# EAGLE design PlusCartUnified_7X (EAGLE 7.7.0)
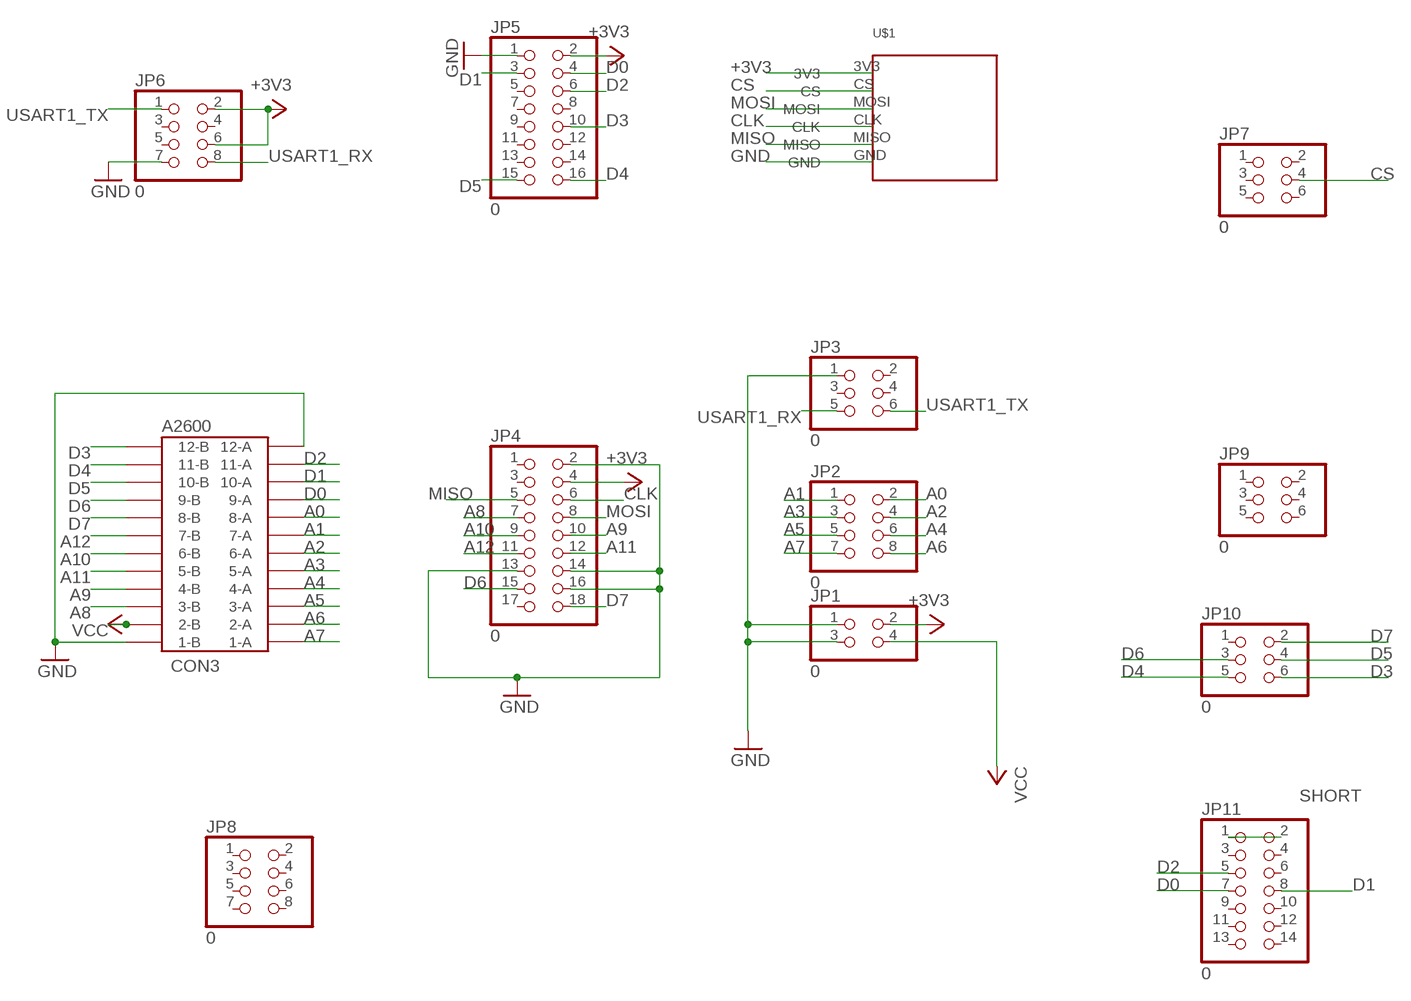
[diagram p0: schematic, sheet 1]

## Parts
CON3  A2600  24PINEDGE-254MM  [24PINEDGE-254MM]
JP1  0  PINHD-2X2  [2X02]
JP2  0  PINHD-2X4  [2X04]
JP3  0  PINHD-2X3  [2X03]
JP4  0  PINHD-2X9  [2X09]
JP5  0  PINHD-2X8  [2X08]
JP6  0  PINHD-2X4  [2X04]
JP7  0  PINHD-2X3  [2X03]
JP8  0  PINHD-2X4  [2X04]
JP9  0  PINHD-2X3  [2X03]
JP10  0  PINHD-2X3  [2X03]
JP11  0  PINHD-2X7  [2X07]
U$1  MICROSD2MICROSD2  [MICROSD_FOOTPRINT]

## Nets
+3V3: JP1.2 JP4.4 JP5.2 JP6.2 JP6.6 U$1.3V3
A0: CON3.8-A JP2.2
A1: CON3.7-A JP2.1
A2: CON3.6-A JP2.4
A3: CON3.5-A JP2.3
A4: CON3.4-A JP2.6
A5: CON3.3-A JP2.5
A6: CON3.2-A JP2.8
A7: CON3.1-A JP2.7
A8: CON3.3-B JP4.7
A9: CON3.4-B JP4.10
A10: CON3.6-B JP4.9
A11: CON3.5-B JP4.12
A12: CON3.7-B JP4.11
CLK: JP4.6 U$1.CLK
CS: JP7.4 U$1.CS
D0: CON3.9-A JP5.4 JP11.7
D1: CON3.10-A JP5.3 JP11.8
D2: CON3.11-A JP5.6 JP11.5
D3: CON3.12-B JP5.10 JP10.6
D4: CON3.11-B JP5.16 JP10.5
D5: CON3.10-B JP5.15 JP10.4
D6: CON3.9-B JP4.15 JP10.3
D7: CON3.8-B JP4.18 JP10.2
GND: CON3.1-B CON3.12-A JP1.1 JP1.3 JP3.1 JP4.2 JP4.13 JP4.14 JP4.16 JP5.1 JP6.7 U$1.GND
MISO: JP4.5 U$1.MISO
MOSI: JP4.8 U$1.MOSI
SHORT: JP11.1 JP11.2
USART1_RX: JP3.5 JP6.8
USART1_TX: JP3.6 JP6.1
VCC: CON3.2-B JP1.4
Unconnected: JP3.2 JP3.3 JP3.4 JP4.1 JP4.3 JP4.17 JP5.5 JP5.7 JP5.8 JP5.9 JP5.11 JP5.12 JP5.13 JP5.14 JP6.3 JP6.4 JP6.5 JP7.1 JP7.2 JP7.3 JP7.5 JP7.6 JP8.1 JP8.2 JP8.3 JP8.4 JP8.5 JP8.6 JP8.7 JP8.8 JP9.1 JP9.2 JP9.3 JP9.4 JP9.5 JP9.6 JP10.1 JP11.3 JP11.4 JP11.6 JP11.9 JP11.10 JP11.11 JP11.12 JP11.13 JP11.14

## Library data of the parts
CON3 = con-edge:24PINEDGE-254MM: 24 PIN EDGE CONNECTOR 2.54mm ATARI 2600 CARTRIDGE PORT
JP1 = pinhead:PINHD-2X2: PIN HEADER
JP2 JP6 = pinhead:PINHD-2X4: PIN HEADER
JP3 = pinhead:PINHD-2X3: PIN HEADER
JP4 = pinhead:PINHD-2X9: PIN HEADER
JP5 = pinhead:PINHD-2X8: PIN HEADER
JP7 JP9 JP10 = pinhead@1:PINHD-2X3: PIN HEADER
JP8 = pinhead@1:PINHD-2X4: PIN HEADER
JP11 = pinhead@1:PINHD-2X7: PIN HEADER
U$1 = MICROSD:MICROSD2

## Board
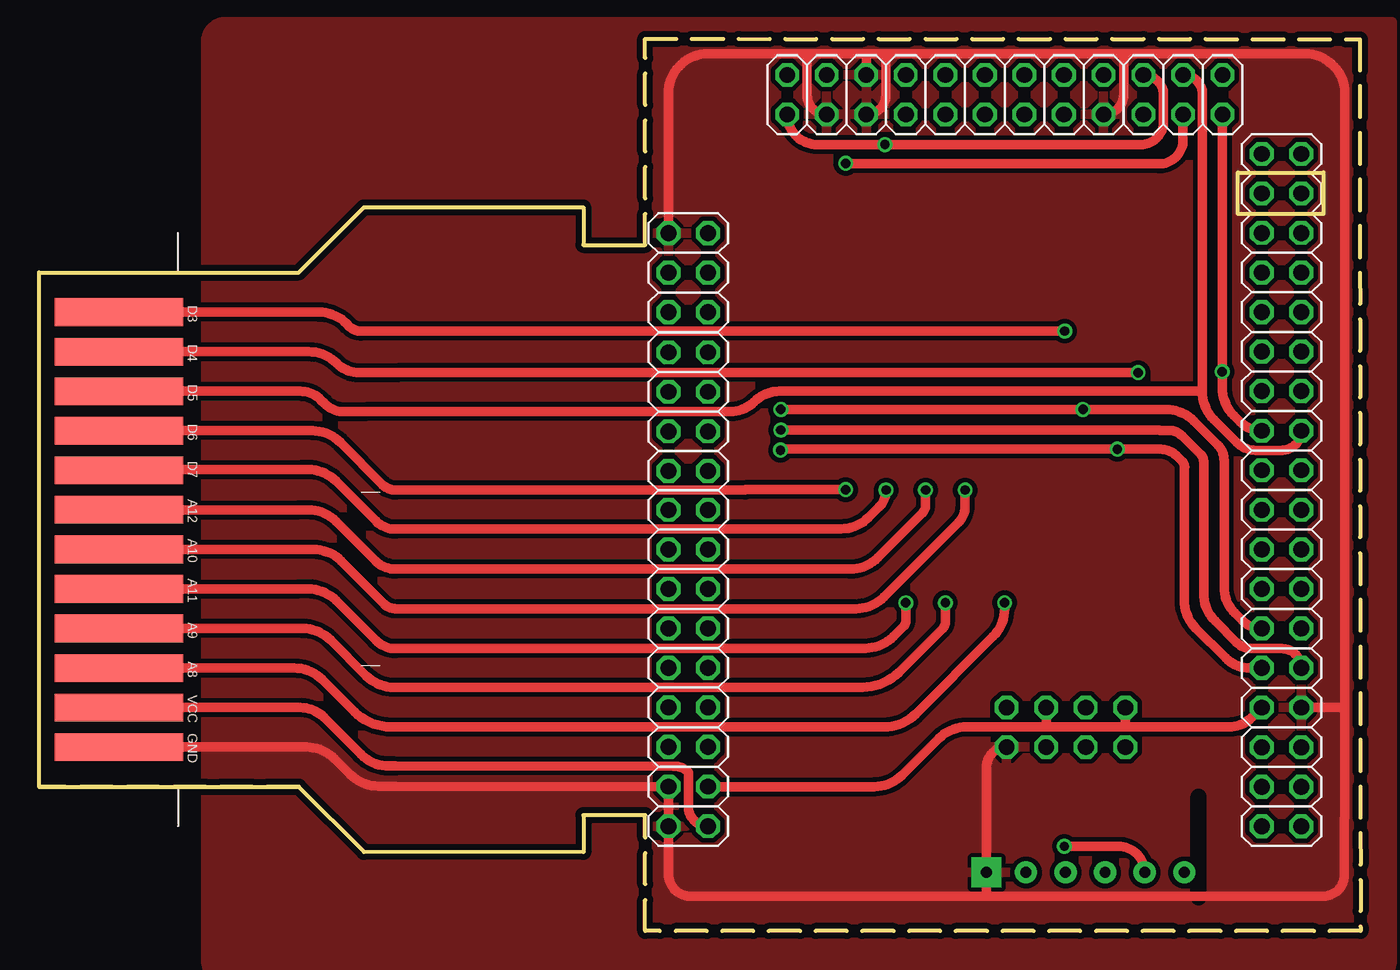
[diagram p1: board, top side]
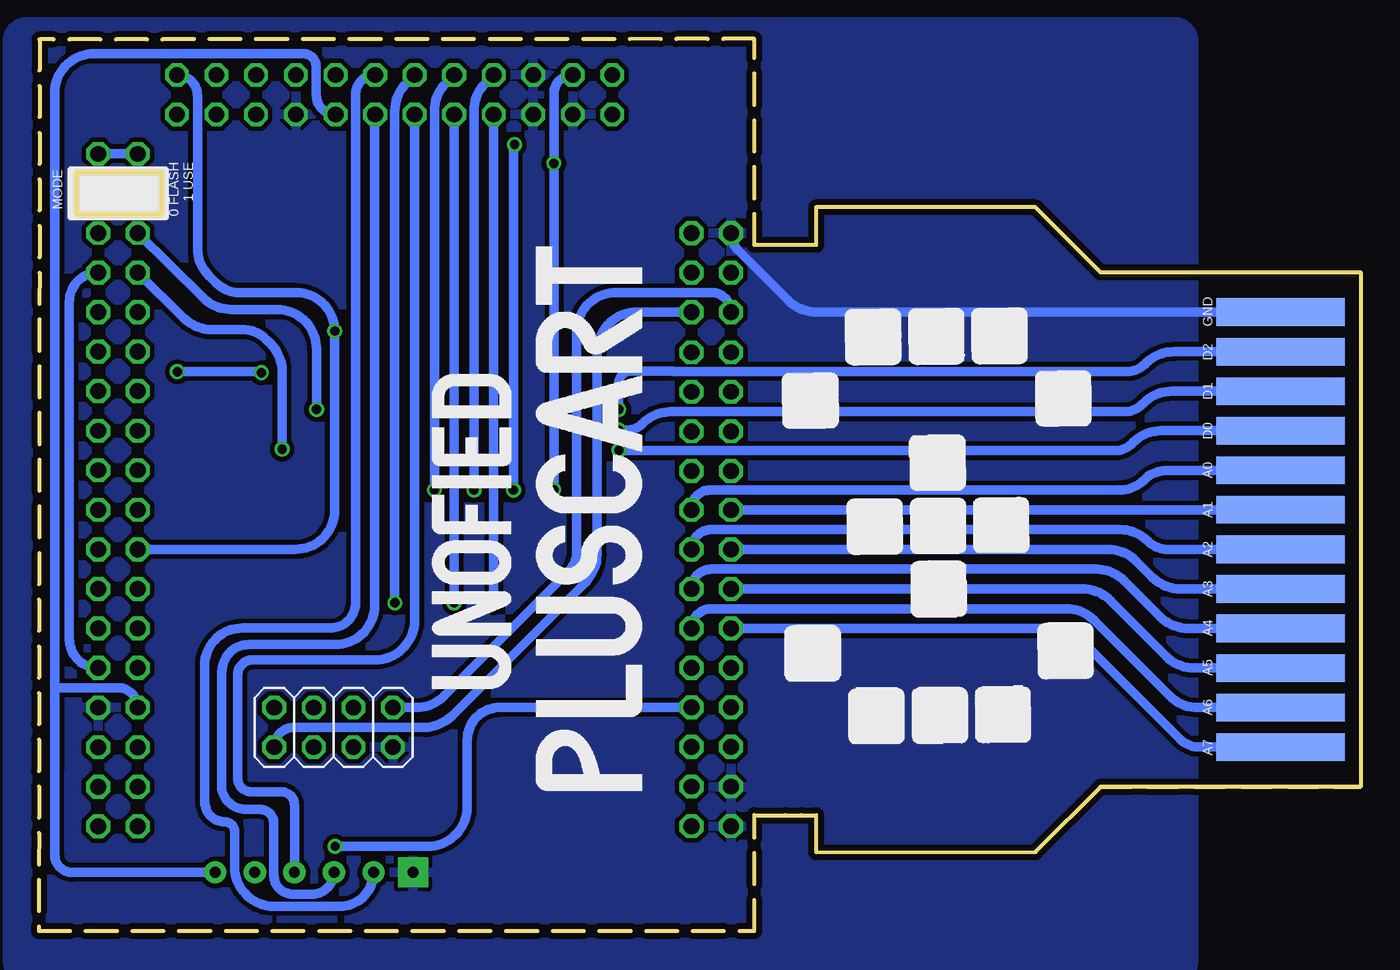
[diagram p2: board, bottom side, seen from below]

Size 84.89 x 57.3 mm. Coordinates in mm from the lower left corner, seen from the top.
Outline: 38.94,7.44 34.98,7.44
Outline: 34.98,7.44 34.98,5.05 20.88,5.08 16.69,9.27
Outline: 0,9.27 0,42.29 16.69,42.29 20.88,46.48 34.98,46.48 34.98,44.07 38.94,44.07 38.94,57.3 84.84,57.28 84.89,0 38.94,0 38.94,7.44
Outline: 0,9.27 16.69,9.27
Outline: 38.94,7.44 34.98,7.44
Outline: 16.69,9.27 0,9.27
Copper layers (1*16): Top 0.0356mm / dielectric 1.5011mm / Bottom 0.0356mm
Design rules "OSHPark2layer": minimum track width 6mil, minimum drill 13mil, track to track 6mil, track to pad 6mil, pad to pad 6mil, via to via 6mil, smd to smd 6mil, copper to edge 15mil, drill to drill 6mil, minimum pad ring 7mil, minimum via ring 7mil, stop-mask expansion 3mil, vias tented up to drill 0mil, thermal gap 10mil
tRestrict: area 74.5,2.2 to 74.5,8.6
Milling: 4 lines

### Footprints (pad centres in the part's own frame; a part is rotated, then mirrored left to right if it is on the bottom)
24PINEDGE-254MM = smd 1.778 x 8.255: 1-A -22.86,-7.62; 2-A -20.32,-7.62; 3-A -17.78,-7.62; 4-A -15.24,-7.62; 5-A -12.7,-7.62; 6-A -10.16,-7.62; 7-A -7.62,-7.62; 8-A -5.08,-7.62; 9-A -2.54,-7.62; 10-A 0,-7.62; 11-A 2.54,-7.62; 12-A 5.08,-7.62 | smd 1.778 x 8.255 bottom: 1-B -22.86,-7.62; 2-B -20.32,-7.62; 3-B -17.78,-7.62; 4-B -15.24,-7.62; 5-B -12.7,-7.62; 6-B -10.16,-7.62; 7-B -7.62,-7.62; 8-B -5.08,-7.62; 9-B -2.54,-7.62; 10-B 0,-7.62; 11-B 2.54,-7.62; 12-B 5.08,-7.62
2X02 = drill 1.016 octagon: 1 -1.27,-1.27; 2 -1.27,1.27; 3 1.27,-1.27; 4 1.27,1.27
2X04 = drill 1.016 octagon: 1 -3.81,-1.27; 2 -3.81,1.27; 3 -1.27,-1.27; 4 -1.27,1.27; 5 1.27,-1.27; 6 1.27,1.27; 7 3.81,-1.27; 8 3.81,1.27
2X03 = drill 1.016 octagon: 1 -2.54,-1.27; 2 -2.54,1.27; 3 0,-1.27; 4 0,1.27; 5 2.54,-1.27; 6 2.54,1.27
2X09 = drill 1.016 octagon: 1 -10.16,-1.27; 2 -10.16,1.27; 3 -7.62,-1.27; 4 -7.62,1.27; 5 -5.08,-1.27; 6 -5.08,1.27; 7 -2.54,-1.27; 8 -2.54,1.27; 9 0,-1.27; 10 0,1.27; 11 2.54,-1.27; 12 2.54,1.27; 13 5.08,-1.27; 14 5.08,1.27; 15 7.62,-1.27; 16 7.62,1.27; 17 10.16,-1.27; 18 10.16,1.27
2X08 = drill 1.016 octagon: 1 -8.89,-1.27; 2 -8.89,1.27; 3 -6.35,-1.27; 4 -6.35,1.27; 5 -3.81,-1.27; 6 -3.81,1.27; 7 -1.27,-1.27; 8 -1.27,1.27; 9 1.27,-1.27; 10 1.27,1.27; 11 3.81,-1.27; 12 3.81,1.27; 13 6.35,-1.27; 14 6.35,1.27; 15 8.89,-1.27; 16 8.89,1.27
2X07 = drill 1.016 octagon: 1 -7.62,-1.27; 2 -7.62,1.27; 3 -5.08,-1.27; 4 -5.08,1.27; 5 -2.54,-1.27; 6 -2.54,1.27; 7 0,-1.27; 8 0,1.27; 9 2.54,-1.27; 10 2.54,1.27; 11 5.08,-1.27; 12 5.08,1.27; 13 7.62,-1.27; 14 7.62,1.27
MICROSD_FOOTPRINT = drill 0.7 pad 1.422: 3V3 -13.97,6.35; CLK -13.97,-1.27; CS -13.97,3.81; MISO -13.97,-3.81; MOSI -13.97,1.27 | drill 0.7 pad 1.93 square: GND -13.97,-6.35

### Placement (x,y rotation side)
CON3  12.75,34.67 90 bottom
JP1  41.71,8 270 top
JP2  41.71,23.24 270 top
JP3  41.71,42.29 270 top
JP4  58.22,53.72 180 top
JP5  79.81,23.24 90 top
JP6  65.96,13.08 0 bottom
JP7  41.71,14.36 270 top
JP8  41.71,33.36 270 top
JP9  79.81,9.26 270 top
JP10  73.48,53.72 0 top
JP11  79.81,42.3 270 top
U$1  67.21,-10.21 270 top

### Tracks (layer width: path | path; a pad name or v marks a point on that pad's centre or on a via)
+3V3
  Top 0.61: JP1.2 53.66,9.27 arc45 55.44,10.01 57.8,12.36 arc-45 59.59,13.11 64.67,13.11 | 64.67,13.11 69.77,13.11 | 69.77,13.11 76.43,13.11 arc45 77.9,13.72 JP5.2 | JP6.2 69.77,13.11 | JP6.6 64.69,13.17 arc-45 64.67,13.11
  Bottom 0.61: JP4.4 arc90 67.07,53.68 67.07,55.5 arc-90 67.94,56.36 81.33,56.36 arc-90 83.87,53.83 83.87,15.62 | 83.87,15.62 83.87,10.37 arc90 83.87,10.36 83.87,4.9 arc-90 82.73,3.76 U$1.3V3 | JP5.2 arc-90 79.81,15.62 83.87,15.62
A0
  Bottom 0.61: JP2.2 42.98,27.12 arc90 41.77,28.33 15.47,28.33 arc-45 13.89,28.98 arc45 12.42,29.59 CON3.8-A
A1
  Bottom 0.61: JP2.1 CON3.7-A
A2
  Bottom 0.61: JP2.4 arc90 41.71,25.78 15.45,25.78 arc45 13.66,25.04 arc-45 12.39,24.51 CON3.6-A
A3
  Bottom 0.61: JP2.3 16.22,24.51 arc45 14.42,23.77 13.37,22.71 arc-45 11.57,21.97 CON3.5-A
A4
  Bottom 0.61: JP2.6 arc90 41.71,23.24 16.98,23.24 arc45 15.18,22.5 12.86,20.18 arc-45 11.06,19.43 CON3.4-A
A5
  Bottom 0.61: JP2.5 17.87,21.97 arc45 16.07,21.23 12.48,17.63 arc-45 10.68,16.89 CON3.3-A
A6
  Bottom 0.61: JP2.8 arc90 41.71,20.7 18.91,20.7 arc45 17.11,19.96 12.25,15.1 arc-45 10.45,14.35 CON3.2-A
A7
  Bottom 0.61: JP2.7 19.75,19.43 arc45 17.95,18.69 11.58,12.32 arc-45 10.36,11.81 CON3.1-A
A8  (via drill 0.6)
  Top 0.61: CON3.3-B 16.4,16.89 arc-45 18.19,16.15 20.26,14.08 arc45 22.6,13.11 54.28,13.11 arc45 56.32,13.95 61.28,18.92 arc45 62.03,20.71 v62.03,21.08
  Bottom 0.61: JP4.7 61.28,54.47 arc-45 62.03,52.67 v62.03,21.08
A9  (via drill 0.6)
  Top 0.61: v58.22,21.08 58.22,19.84 arc-45 58.05,19.45 55.23,16.62 arc-45 52.89,15.65 22.91,15.65 22.82,15.65 arc-45 21.02,16.39 18.73,18.69 arc45 16.93,19.43 CON3.4-B
  Bottom 0.61: JP4.10 v58.22,21.08
A10  (via drill 0.6)
  Top 0.61: v59.49,28.32 59.49,27.28 arc-45 59.06,26.24 54.26,21.45 arc-45 52.47,20.7 22.91,20.7 arc-45 22.17,21.01 19.41,23.77 arc45 17.62,24.51 CON3.6-B
  Bottom 0.61: JP4.9 58.74,54.47 arc-45 59.49,52.67 v59.49,28.32
A11  (via drill 0.6)
  Top 0.61: v55.68,21.08 55.68,19.89 arc-45 55.55,19.59 54.87,18.91 arc-45 53.07,18.16 22.97,18.16 arc45 22.91,18.14 arc-45 21.65,18.66 19.08,21.23 arc45 17.29,21.97 16.7,21.97 CON3.5-B
  Bottom 0.61: JP4.12 v55.68,21.08
A12  (via drill 0.6)
  Top 0.61: v56.95,28.32 56.95,27.33 arc-45 56.75,26.85 53.88,23.98 arc-45 52.08,23.24 22.91,23.24 arc-45 21.61,23.78 19.08,26.31 arc45 17.29,27.05 16.71,27.05 CON3.7-B
  Bottom 0.61: JP4.11 56.2,54.47 arc-45 56.95,52.67 v56.95,28.32
CLK
  Bottom 0.61: JP4.6 arc-45 63.32,52.4 63.32,20.94 arc90 65.86,18.39 71.42,18.39 arc-90 73.11,16.7 arc-90 73.16,16.65 73.16,9.39 arc-90 71.59,7.81 70.68,7.81 arc90 69.8,6.93 69.8,3.58 arc-90 68.58,2.36 67.34,2.36 arc-90 U$1.CLK
CS  (via drill 0.6)
  Top 0.61: v65.86,5.44 69.34,5.44 arc-90 U$1.CS
  Bottom 0.61: JP7.4 55.28,14.36 arc-90 57.38,12.26 57.38,7.98 arc90 59.92,5.44 v65.86,5.44
D0  (via drill 0.6)
  Top 0.61: v47.62,30.89 47.68,30.95 v69.27,30.95 72.05,30.95 arc-45 73.05,30.53 73.44,30.14 arc-45 73.58,29.79 arc45 73.56,29.73 73.56,21.24 arc45 74.3,19.45 76.23,17.53 arc45 77.76,16.89 JP5.4
  Bottom 0.61: v47.62,30.89 47.59,30.85 15.77,30.85 arc-45 14.71,31.29 14.61,31.39 arc45 12.82,32.13 CON3.9-A | v69.27,30.95 69.27,35.93 arc-45 70.01,37.73 70.28,38 arc-45 71.81,38.63 73.79,38.63 arc45 75.58,39.38 JP11.7
D1  (via drill 0.6)
  Top 0.61: JP5.3 arc90 79.83,18.14 77.9,18.14 arc-45 76.9,18.55 75.55,19.91 arc-45 74.8,21.7 74.8,30.18 arc45 74.62,30.61 73.43,31.8 arc45 72.57,32.16 72.01,32.16 arc-45 71.95,32.18 v47.65,32.18
  Bottom 0.61: JP5.3 arc90 82.93,18.74 82.93,40.41 arc90 JP11.8 | CON3.10-A 12.13,34.67 arc-45 13.93,33.93 14.02,33.83 arc45 15.19,33.35 44.31,33.35 arc-45 46.11,32.61 46.18,32.54 arc45 47.04,32.18 v47.65,32.18
D2  (via drill 0.6)
  Top 0.61: v47.65,33.5 v67.06,33.5 72.38,33.5 arc-45 74.18,32.76 75.72,31.22 arc-45 76.12,30.23 76.12,22.08 arc45 76.81,20.42 77.28,19.95 arc45 JP5.6
  Bottom 0.61: JP11.5 74.34,40.67 arc-45 72.54,39.93 69.6,39.93 arc90 67.06,37.39 v67.06,33.5 | v47.65,33.5 47.65,35.18 arc90 46.86,35.97 44.18,35.97 arc90 44.16,35.94 14.97,35.94 arc-45 13.87,36.4 13.8,36.47 arc45 12,37.21 CON3.11-A
D3  (via drill 0.6)
  Top 0.61: v65.89,38.53 20.67,38.53 arc-45 19.94,38.84 19.77,39.01 arc45 17.97,39.75 CON3.12-B
  Bottom 0.61: JP5.10 68.42,24.51 arc-90 65.88,27.05 65.88,38.51 arc-45 v65.89,38.53 arc-90 68.36,41 72.03,41 arc45 73.49,41.61 73.96,42.08 arc45 74.7,43.88 74.7,53.66 arc-90 JP10.6
D4  (via drill 0.6)
  Top 0.61: JP5.16 arc-45 77.15,32.71 76.74,33.11 arc-45 76,34.91 v76,35.93 arc45 76.02,35.98 JP10.5 | v70.6,35.86 23.04,35.86 20.58,35.86 arc-45 19.15,36.45 19.13,36.47 arc45 17.34,37.21 CON3.11-B
  Bottom 0.61: v70.6,35.86 arc-45 70.77,35.93 v76,35.93
D5
  Top 0.61: JP5.15 arc-90 79.82,30.88 78.16,30.88 arc-45 76.95,31.38 75.46,32.86 arc-45 74.71,34.66 74.71,34.67 | JP10.4 arc-90 74.73,53.74 74.73,34.69 arc-90 74.71,34.67 | 74.71,34.67 47.58,34.67 arc45 45.92,33.98 arc-45 44.39,33.35 20.98,33.35 20.65,33.35 19.63,33.35 arc-45 18.34,33.88 18.11,34.11 arc45 16.76,34.67 CON3.10-B
D6  (via drill 0.6)
  Top 0.61: v51.82,28.35 45.39,28.35 45.36,28.32 22.91,28.32 arc-45 22.09,28.66 19.36,31.39 arc45 17.57,32.13 CON3.9-B | JP10.3 73.48,50.81 arc-90 71.95,49.28 51.86,49.28 arc-90 v51.82,49.31
  Bottom 0.61: v51.82,28.35 v51.82,49.31 51.82,53.77 arc90 JP4.15
D7  (via drill 0.6)
  Top 0.61: v54.41,28.32 arc-45 53.96,27.24 53.29,26.57 arc-45 51.51,25.83 22.97,25.83 arc45 22.91,25.81 arc-45 21.65,26.33 19.08,28.9 arc45 17.29,29.64 16.76,29.64 16.38,29.64 5.25,29.64 arc45 CON3.8-B | JP4.18 arc90 49.99,50.52 v54.34,50.52 70.76,50.52 arc90 72.23,51.98 72.23,53.7 arc90 JP10.2
  Bottom 0.61: v54.41,28.32 54.41,50.45 arc-90 v54.34,50.52
GND
  Top 0.61: 83.87,14.45 83.87,7.25 arc90 83.85,7.23 83.85,3.58 arc-90 82.5,2.23 60.71,2.23 | JP5.1 83.77,14.35 arc90 83.87,14.45 | 83.87,14.45 83.87,53.81 arc90 81.33,56.36 69.68,56.36 | 69.68,56.36 54.41,56.36 | 54.41,56.36 53.19,56.36 | JP4.2 arc90 69.68,53.75 69.68,56.36 | JP3.1 40.44,53.81 arc-90 42.98,56.36 49.33,56.36 | 49.33,56.36 53.19,56.36 | JP4.13 53.14,56.3 arc-90 53.19,56.36 | JP4.16 arc-90 49.33,53.72 49.33,56.36 | JP4.14 arc90 54.41,53.72 54.41,56.36 | CON3.1-B 17.18,11.81 arc-45 18.98,11.07 20.01,10.04 arc45 21.8,9.3 22.91,9.3 JP1.1 JP1.3 40.44,3.63 arc90 41.83,2.23 60.71,2.23 | JP6.7 arc90 60.86,10.52 U$1.GND 60.86,2.39 arc-90 60.71,2.23
  Bottom 0.61: JP3.1 arc-45 39.99,43.75 36.74,40.5 arc-45 34.94,39.75 CON3.12-A
  pour Top (isolate 0.305): 10.72,-1.27 10.72,57.15 arc-90 11.99,58.42 86.92,58.42 86.92,-1.91 arc-90 85.65,-3.18 83.74,-3.18 11.99,-3.18 arc-90 10.72,-1.91
  pour Bottom (isolate 0.305): 10.72,57.15 10.72,-1.91 arc90 11.99,-3.18 79.93,-3.18 85.65,-3.18 arc90 86.92,-1.91 86.92,55.25 86.92,57.15 arc90 85.65,58.42 13.89,58.42 11.99,58.42 arc90
MISO
  Bottom 0.61: JP4.5 arc-90 64.55,53.74 64.55,21.09 arc90 66.19,19.45 71.84,19.45 arc-90 74.24,17.05 74.24,8.29 arc-90 72.97,7.02 arc90 72.31,6.36 72.31,4.12 arc-90 69.77,1.58 65.58,1.58 arc-90 U$1.MISO
MOSI
  Bottom 0.61: JP4.8 60.76,19.95 arc90 63.3,17.41 71.17,17.41 arc-90 72.12,16.46 72.12,9.79 arc-90 71.27,8.94 69.32,8.94 arc90 68.48,8.1 U$1.MOSI
SHORT
  Bottom 0.61: JP11.1 JP11.2
USART1_RX
  Bottom 0.61: JP3.5 arc-90 41.71,41.02 47.8,41.02 arc-90 50.34,38.48 50.34,24.38 arc45 50.88,23.08 58.87,15.1 arc45 60.67,14.35 JP6.8
USART1_TX
  Bottom 0.61: JP6.1 arc90 68.5,13.08 60.16,13.08 arc-45 58.36,13.82 49.79,22.39 arc-45 49.05,24.19 arc-45 49.03,24.23 49.03,37.21 arc90 46.49,39.75 JP3.6
VCC
  Top 0.61: JP1.4 arc-90 41.71,8 arc45 41.71,8 41.71,10.2 arc45 40.77,10.59 22.91,10.59 22.49,10.59 arc-45 20.69,11.34 18.32,13.7 arc45 16.76,14.35 CON3.2-B

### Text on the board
tNames: D3 | D4 | D5 | D6 | D7 | A12 | A10 | A11 | A9 | A8 | VCC | GND
bNames: 0 FLASH / 1 USE | MODE | GND | D2 | D1 | D0 | A0 | A1 | A2 | A3 | A4 | A5 | A6 | A7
